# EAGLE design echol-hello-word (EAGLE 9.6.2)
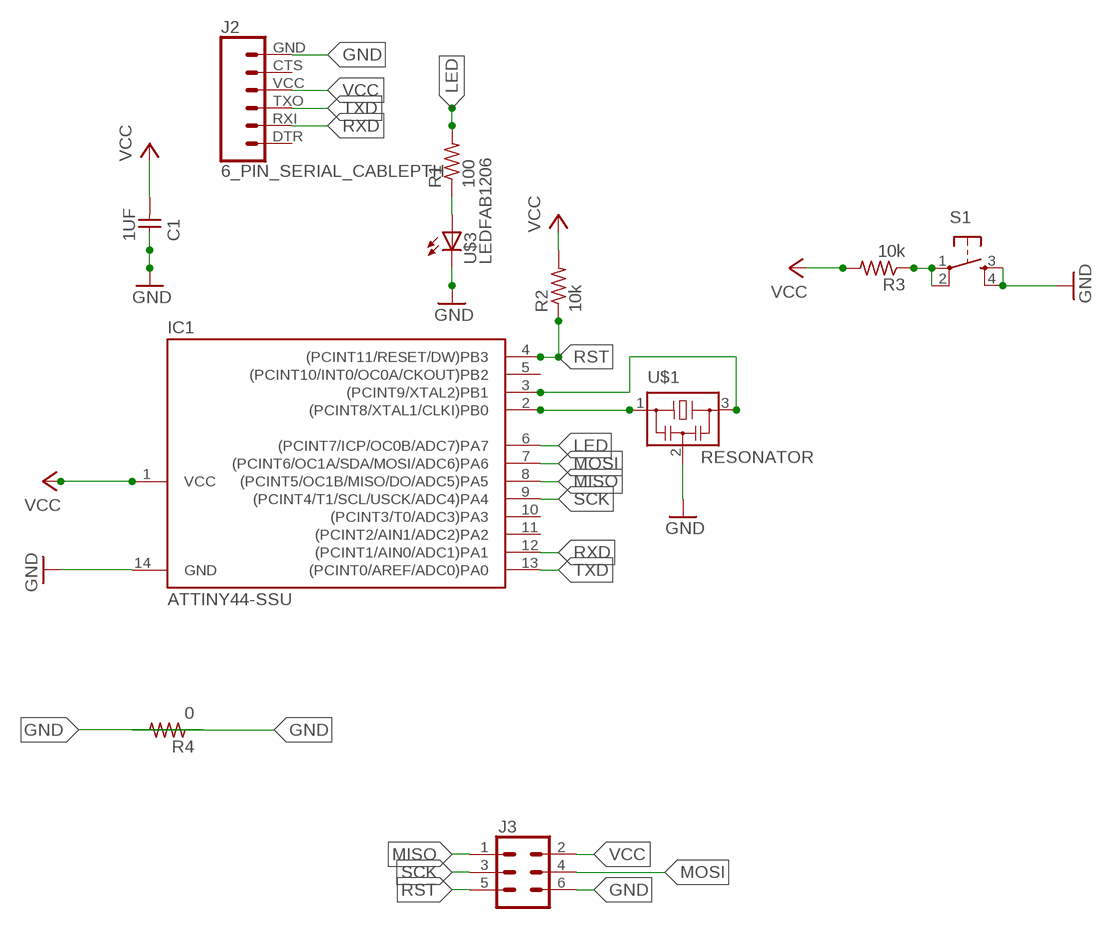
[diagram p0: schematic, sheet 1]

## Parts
C1  1UF  CAP-UNPOLARIZEDFAB  [C1206FAB]
IC1  ATTINY44-SSU  [SOIC14]
J2  6_PIN_SERIAL_CABLEPTH  [FTDI_BASIC]
J3  CONN_03X22X3_SILK_MALE_PTH  [2X3]
R1  100  RES-US1206FAB  [R1206FAB]
R2  10k  RES-US1206FAB  [R1206FAB]
R3  10k  RES-US1206FAB  [R1206FAB]
R4  0  RES-US1206FAB  [R1206FAB]
S1  6MM_SWITCH6MM_SWITCH  [6MM_SWITCH]
U$1  RESONATOR  [EFOBM]
U$3  LEDFAB1206  [LED1206FAB]

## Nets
GND: C1.1 IC1.14(GND) J2.GND J3.6 R4.1 R4.2 S1.3(S) S1.4(S1) U$1.2 U$3.2(C)
LED: IC1.6((PCINT7/ICP/OC0B/ADC7)PA7) R1.2
MISO: IC1.8((PCINT5/OC1B/MISO/DO/ADC5)PA5) J3.1
MOSI: IC1.7((PCINT6/OC1A/SDA/MOSI/ADC6)PA6) J3.4
N$1: R1.1 U$3.1(A)
N$2: IC1.2((PCINT8/XTAL1/CLKI)PB0) U$1.1
N$3: IC1.3((PCINT9/XTAL2)PB1) U$1.3
N$5: R3.1 S1.1(P) S1.2(P1)
RST: IC1.4((PCINT11/RESET/DW)PB3) J3.5 R2.1
RXD: IC1.12((PCINT1/AIN0/ADC1)PA1) J2.RXI
SCK: IC1.9((PCINT4/T1/SCL/USCK/ADC4)PA4) J3.3
TXD: IC1.13((PCINT0/AREF/ADC0)PA0) J2.TXO
VCC: C1.2 IC1.1(VCC) J2.VCC J3.2 R2.2 R3.2
Unconnected: IC1.5((PCINT10/INT0/OC0A/CKOUT)PB2) IC1.10((PCINT3/T0/ADC3)PA3) IC1.11((PCINT2/AIN1/ADC2)PA2) J2.CTS J2.DTR

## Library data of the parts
C1 = fab:CAP-UNPOLARIZED
IC1 = fab:ATTINY44
J2 = SparkFun-Connectors:6_PIN_SERIAL_CABLE: 6-pin header connection for use with the "FTDI BASIC" pinout - CABLE SIDE. Also known as "Arduino Serial Program Header". This is used on a design to provide a 6-pin connection point for serial communication usually from a USB cable (D+/D-) to these headers (RX/TX). It also has the remaining pins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
J3 = SparkFun-Connectors:CONN_03X2: Multi connection point. Often used as Generic Header-pin footprint for 0.1 inch spaced/style header connections You can populate with any combo of single row headers, but if you'd like an exact match, check these: Header - 2x3 (Male, 0.1") (PRT-12807) Header - 2x3 (Female, 0.1") (PRT-13010) 2x3 Pin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; PROD_ID: CONN-09701
R1-R4 = fab:RES-US: Resistor (US Symbol)
S1 = fab:6MM_SWITCH: OMRON SWITCH
U$1 = fab:RESONATOR
U$3 = fab:LED: LED

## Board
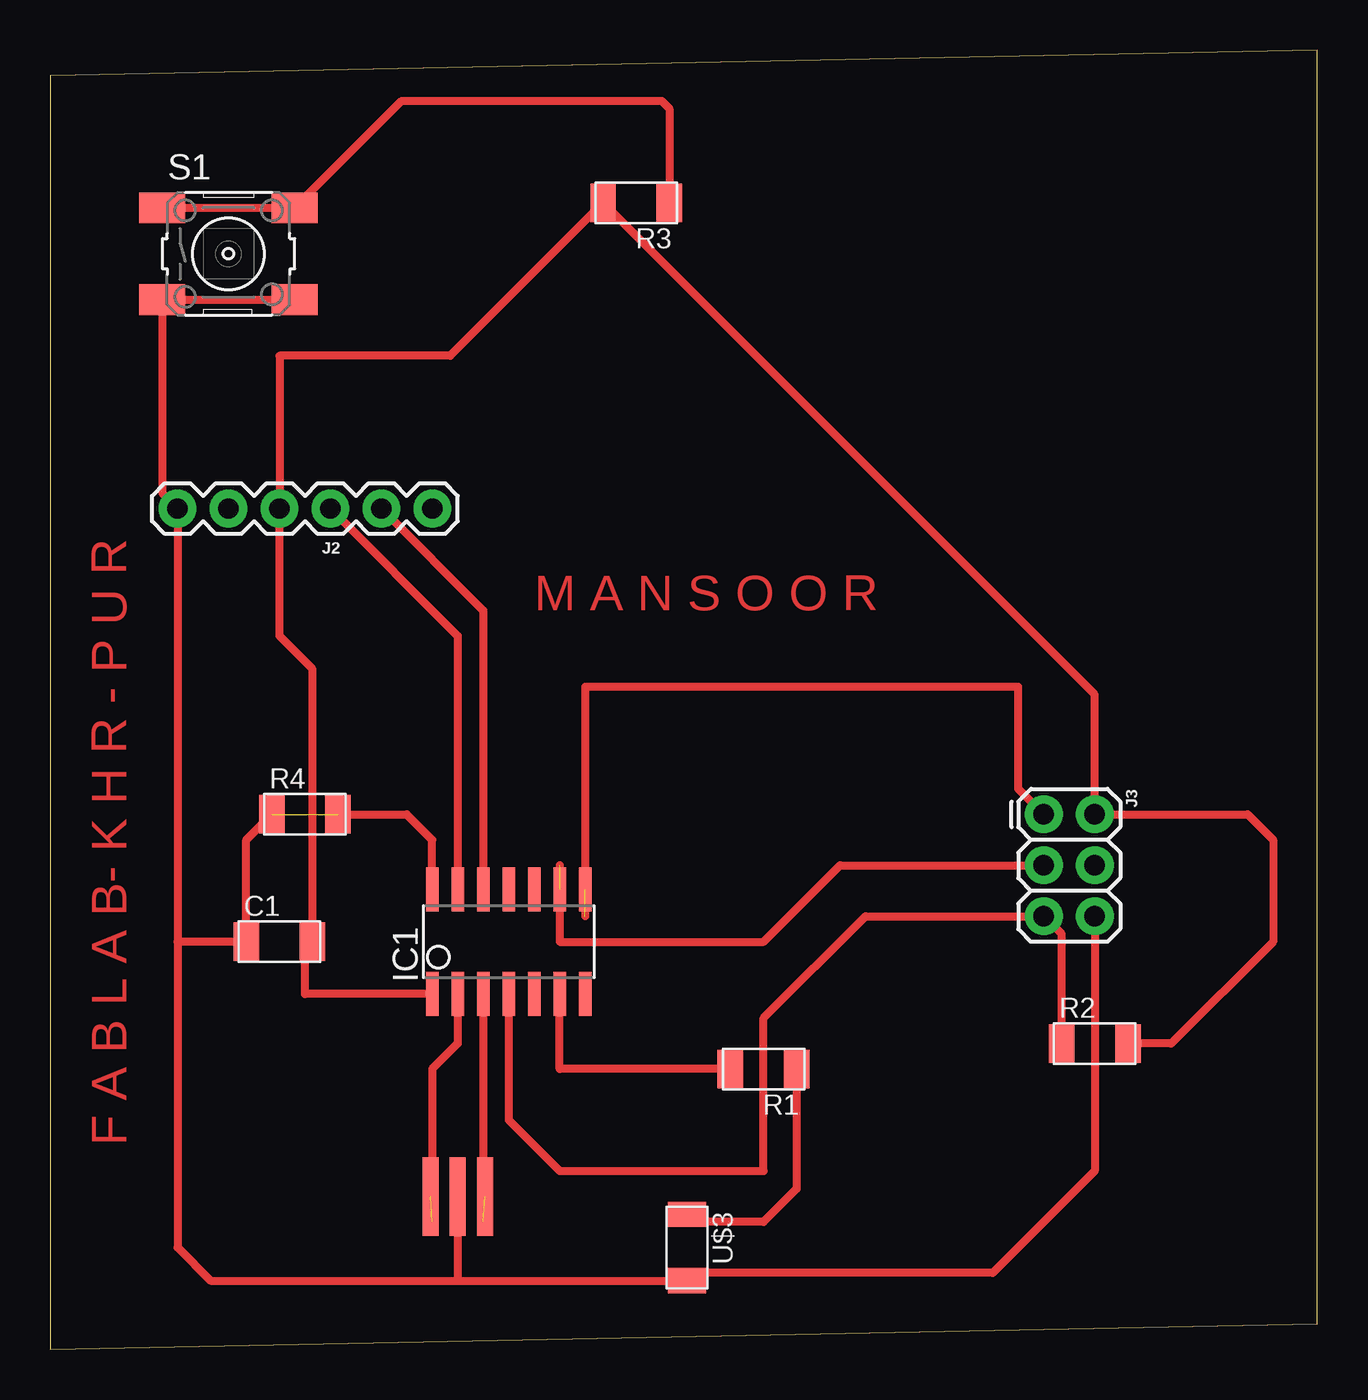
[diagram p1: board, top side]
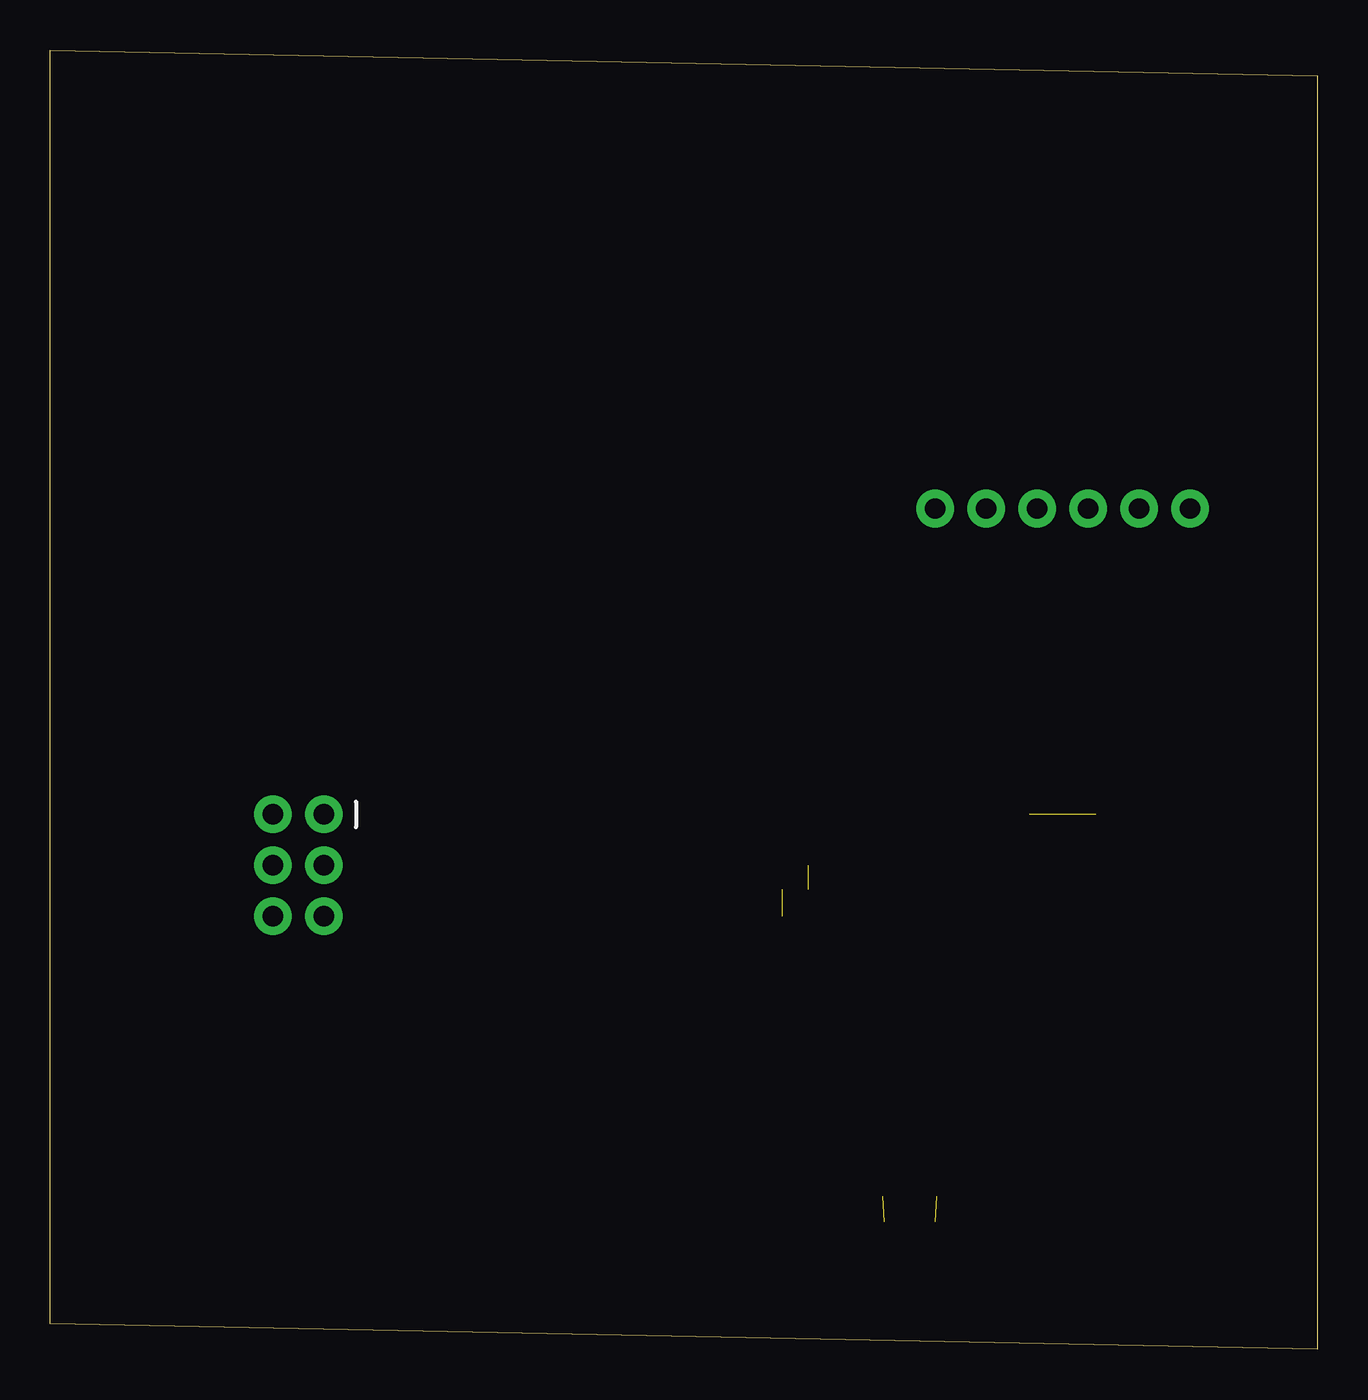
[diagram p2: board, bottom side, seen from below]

Size 63.17 x 64.76 mm. Coordinates in mm from the lower left corner, seen from the top.
Outline: 0,0 63.17,1.27 63.17,64.76 0,63.49 0,0
Copper layers (1*16): Top 0.035mm / dielectric 1.5mm / Bottom 0.035mm
Design rules "default *": minimum track width 6mil, minimum drill 0.35mm, track to track 8mil, track to pad 8mil, pad to pad 8mil, via to via 8mil, smd to smd 8mil, copper to edge 40mil, drill to drill 6mil, minimum pad ring 10mil, minimum via ring 8mil, stop-mask expansion 4mil, vias tented up to drill 0mil, thermal gap 10mil

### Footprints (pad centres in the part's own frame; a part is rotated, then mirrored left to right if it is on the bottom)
C1206FAB = smd 1.27 x 1.905: 1 -1.651,0; 2 1.651,0
SOIC14 = smd 0.61 x 2.21: 1 -3.81,-2.603; 2 -2.54,-2.603; 3 -1.27,-2.603; 4 0,-2.603; 5 1.27,-2.603; 6 2.54,-2.603; 7 3.81,-2.603; 8 3.81,2.603; 9 2.54,2.603; 10 1.27,2.603; 11 0,2.603; 12 -1.27,2.603; 13 -2.54,2.603; 14 -3.81,2.603
FTDI_BASIC = drill 1.016 pad 1.88: CTS 10.16,0; DTR 0,0; GND 12.7,0; RXI 2.54,0; TXO 5.08,0; VCC 7.62,0
2X3 = drill 1.016 pad 1.88: 1 0,0; 2 0,2.54; 3 2.54,0; 4 2.54,2.54; 5 5.08,0; 6 5.08,2.54
R1206FAB = smd 1.27 x 1.905: 1 -1.651,0; 2 1.651,0
6MM_SWITCH = smd 2.286 x 1.524: 1 -3.302,2.286; 2 3.302,2.286; 3 -3.302,-2.286; 4 3.302,-2.286
EFOBM = smd 0.8 x 3.9: 1 -1.35,0; 2 0,0; 3 1.35,0
LED1206FAB = smd 1.27 x 1.905: 1 -1.651,0; 2 1.651,0

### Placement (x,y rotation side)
C1  11.43,20.32 0 top
IC1  22.86,20.32 0 top
J2  19.05,41.91 180 top
J3  49.53,26.67 270 top
R1  35.56,13.97 180 top
R2  52.07,15.24 0 top
R3  29.21,57.15 180 top
R4  12.7,26.67 0 top
S1  8.89,54.61 0 top
U$1  20.32,7.62 0 top
U$3  31.75,5.08 270 top

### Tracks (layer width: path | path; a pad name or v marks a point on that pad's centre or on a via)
GND  (1 unrouted)
  Top 0.406: 20.32,3.43 U$3.2 32.13,3.81 46.99,3.81 52.07,8.89 J3.6 | U$1.2 20.32,3.43 | S1.4 S1.3 5.59,42.67 J2.GND 6.35,20.32 | 20.32,3.43 8,3.43 6.35,5.08 6.35,20.32 | 6.35,20.32 C1.1 9.78,25.4 R4.1 | R4.2 17.78,26.67 19.05,25.4 IC1.14
LED
  Top 0.406: R1.2 25.4,13.97 IC1.6
MISO  (1 unrouted)
  Top 0.406: J3.1 48.26,27.94 48.26,33.02 26.67,33.02 26.67,21.59
N$1
  Top 0.406: R1.1 37.21,8 35.56,6.35 32.13,6.35 U$3.1
N$2  (1 unrouted)
  Top 0.406: IC1.2 20.32,15.24 19.05,13.97 19.05,6.35
N$3  (1 unrouted)
  Top 0.406: 21.53,17.78 IC1.3 21.59,6.35
N$5
  Top 0.406: S1.1 S1.2 17.53,62.23 30.48,62.23 30.86,61.85 R3.1
RST
  Top 0.406: 22.86,12.7 IC1.4 22.86,11.43 25.4,8.89 35.56,8.89 35.56,16.51 40.64,21.59 J3.5 50.42,20.7 R2.1
RXD
  Top 0.406: J2.RXI 21.59,36.83 IC1.12
SCK  (1 unrouted)
  Top 0.406: 25.4,24.13 25.4,20.32 35.56,20.32 39.37,24.13 J3.3
TXD
  Top 0.406: J2.TXO 20.32,35.56 IC1.13
VCC
  Top 0.406: R2.2 55.88,15.24 60.96,20.32 60.96,25.4 59.69,26.67 J3.2 52.07,32.64 R3.2 19.94,49.53 11.43,49.53 J2.VCC 11.43,35.56 13.08,33.91 C1.2 12.7,19.94 12.7,17.72 IC1.1

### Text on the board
Top: M A N S O O R | F A B L A B- K H R - P U R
